|   stm32f427_437_429_439_lqfp208 IBIS Model
[IBIS ver]   4.2
[File name]  stm32f427_437_429_439_lqfp208.ibs
[File Rev]   1.3
[Date]   05-30-2014
[Source] Data Created at STMicroelectronics
[Notes]   File originated from ELDO simulations.
[Disclaimer]  This information is for modeling purpose only and is
   not guaranted. The information is subject to change without
   notice.
[Copyright] Copyright 2014 STMicroelectronics Inc.
[Component] stm32f427_437_429_439_lqfp208
[Manufacturer] STMicroelectronics
[Package]
| variable   typ   min   max
R_pkg   0.0   NA   NA
L_pkg   0.0H   NA   NA
C_pkg   0.0F   NA   NA
[Pin]   signal_name   model_name   R_pin   L_pin   C_pin
1   PE2   io8p_arsudq_ft   282.4E-3   13.6E-9   386.2E-15
2   PE3   io8p_arsudq_ft   277.3E-3   13.3E-9   362.7E-15
3   PE4   io8p_arsudq_ft   272.4E-3   13.0E-9   340.3E-15
4   PE5   io8p_arsudq_ft   267.8E-3   12.7E-9   318.8E-15
5   PE6   io8p_arsudq_ft   263.3E-3   12.4E-9   298.2E-15
6   VBAT   POWER   259.0E-3   12.1E-9   278.6E-15
7   PI8   io8p_arsudq_ft_v33   254.9E-3   11.9E-9   260.0E-15
8   PC13   io8p_arwsudq_ft_v33   251.1E-3   11.6E-9   242.3E-15
9   PC14   io8p_arwsudq_ft   247.4E-3   11.4E-9   225.6E-15
10   PC15   io8p_arsudq_ft   244.0E-3   11.2E-9   209.8E-15
11   PI9   io8p_arsudq_ft   240.8E-3   11.0E-9   195.0E-15
12   PI10   io8p_arsudq_ft   237.8E-3   10.8E-9   181.1E-15
13   PI11   io8p_arsudq_ft   234.9E-3   10.6E-9   168.2E-15
14   VSS   GND   232.3E-3   10.5E-9   156.3E-15
15   VDD   POWER   229.9E-3   10.3E-9   145.3E-15
16   PF0   io8p_arsudq_i2cin_ft   227.8E-3   10.2E-9   135.3E-15
17   PF1   io8p_arsudq_i2cin_ft   225.8E-3   10.1E-9   126.2E-15
18   PF2   io8p_arsudq_ft   224.0E-3   9.9E-9   118.1E-15
19   PI12   io8p_arsudq_ft   222.4E-3   9.9E-9   110.9E-15
20   PI13   io8p_arsudq_ft   221.1E-3   9.8E-9   104.7E-15
21   PI14   io8p_arsudq_ft   219.9E-3   9.7E-9   99.4E-15
22   PF3   io8p_arwsudq_ft   219.0E-3   9.6E-9   95.1E-15
23   PF4   io8p_arwsudq_ft   218.3E-3   9.6E-9   91.8E-15
24   PF5   io8p_arwsudq_ft   217.8E-3   9.6E-9   89.4E-15
25   VSS   GND   217.4E-3   9.5E-9   87.9E-15
26   VDD   POWER   217.3E-3   9.5E-9   87.5E-15
27   PF6   io8p_arwsudq_ft   217.3E-3   9.5E-9   87.5E-15
28   PF7   io8p_arwsudq_ft   217.4E-3   9.5E-9   87.9E-15
29   PF8   io8p_arwsudq_ft   217.8E-3   9.6E-9   89.4E-15
30   PF9   io8p_arwsudq_ft   218.3E-3   9.6E-9   91.8E-15
31   PF10   io8p_arwsudq_ft   219.0E-3   9.6E-9   95.1E-15
32   PH0   io8p_arsudq_ft   219.9E-3   9.7E-9   99.4E-15
33   PH1   io8p_arsudq_ft   221.1E-3   9.8E-9   104.7E-15
34   NRST   ioreset_ft_v33   222.4E-3   9.9E-9   110.9E-15
35   PC0   io8p_ar3wsudq_ft   224.0E-3   9.9E-9   118.1E-15
36   PC1   io8p_ar3wsudq_ft   225.8E-3   10.1E-9   126.2E-15
37   PC2   io8p_ar3wsudq_ft   227.8E-3   10.2E-9   135.3E-15
38   PC3   io8p_ar3wsudq_ft   229.9E-3   10.3E-9   145.3E-15
39   VDD   POWER   232.3E-3   10.5E-9   156.3E-15
40   VREFM   POWER   234.9E-3   10.6E-9   168.2E-15
41   VREFP   POWER   237.8E-3   10.8E-9   181.1E-15
42   VDDA   POWER   240.8E-3   11.0E-9   195.0E-15
43   PA0   io8p_ar3wsudq_ft_v33   244.0E-3   11.2E-9   209.8E-15
44   PA1   io8p_ar3wsudq_ft   247.4E-3   11.4E-9   225.6E-15
45   PA2   io8p_ar3wsudq_ft   251.1E-3   11.6E-9   242.3E-15
46   PH2   io8p_arsudq_ft   254.9E-3   11.9E-9   260.0E-15
47   PH3   io8p_arsudq_ft   259.0E-3   12.1E-9   278.6E-15
48   PH4   io8p_arsudq_i2cin_ft   263.3E-3   12.4E-9   298.2E-15
49   PH5   io8p_arsudq_i2cin_ft   267.8E-3   12.7E-9   318.8E-15
50   PA3   io8p_ar3wsudq_ft   272.4E-3   13.0E-9   340.3E-15
51   VSS   GND   277.3E-3   13.3E-9   362.7E-15
52   VDD   POWER   282.4E-3   13.6E-9   386.2E-15
53   PA4   io8p_ar3wsudq_ft   282.4E-3   13.6E-9   386.2E-15
54   PA5   io8p_ar3wsudq_ft   277.3E-3   13.3E-9   362.7E-15
55   PA6   io8p_ar3wsudq_ft   272.4E-3   13.0E-9   340.3E-15
56   PA7   io8p_ar3wsudq_ft   267.8E-3   12.7E-9   318.8E-15
57   PC4   io8p_ar3wsudq_ft   263.3E-3   12.4E-9   298.2E-15
58   PC5   io8p_ar3wsudq_ft   259.0E-3   12.1E-9   278.6E-15
59   VDD   POWER   254.9E-3   11.9E-9   260.0E-15
60   VSS   GND   251.1E-3   11.6E-9   242.3E-15
61   PB0   io8p_ar3wsudq_ft   247.4E-3   11.4E-9   225.6E-15
62   PB1   io8p_ar3wsudq_ft   244.0E-3   11.2E-9   209.8E-15
63   PB2   io8p_ar3wsudq_ft   240.8E-3   11.0E-9   195.0E-15
64   PI15   io8p_arsudq_ft   237.8E-3   10.8E-9   181.1E-15
65   PJ0   io8p_arsudq_ft   234.9E-3   10.6E-9   168.2E-15
66   PJ1   io8p_arsudq_ft   232.3E-3   10.5E-9   156.3E-15
67   PJ2   io8p_arsudq_ft   229.9E-3   10.3E-9   145.3E-15
68   PJ3   io8p_arsudq_ft   227.8E-3   10.2E-9   135.3E-15
69   PJ4   io8p_arsudq_ft   225.8E-3   10.1E-9   126.2E-15
70   PF11   io8p_arsudq_ft   224.0E-3   9.9E-9   118.1E-15
71   PF12   io8p_arsudq_ft   222.4E-3   9.9E-9   110.9E-15
72   VSS   GND   221.1E-3   9.8E-9   104.7E-15
73   VDD   POWER   219.9E-3   9.7E-9   99.4E-15
74   PF13   io8p_arsudq_ft   219.0E-3   9.6E-9   95.1E-15
75   PF14   io8p_arsudq_ft   218.3E-3   9.6E-9   91.8E-15
76   PF15   io8p_arsudq_ft   217.8E-3   9.6E-9   89.4E-15
77   PG0   io8p_arsudq_ft   217.4E-3   9.5E-9   87.9E-15
78   PG1   io8p_arsudq_ft   217.3E-3   9.5E-9   87.5E-15
79   PE7   io8p_arsudq_ft   217.3E-3   9.5E-9   87.5E-15
80   PE8   io8p_arsudq_ft   217.4E-3   9.5E-9   87.9E-15
81   PE9   io8p_arsudq_ft   217.8E-3   9.6E-9   89.4E-15
82   VSS   GND   218.3E-3   9.6E-9   91.8E-15
83   VDD   POWER   219.0E-3   9.6E-9   95.1E-15
84   PE10   io8p_arsudq_ft   219.9E-3   9.7E-9   99.4E-15
85   PE11   io8p_arsudq_ft   221.1E-3   9.8E-9   104.7E-15
86   PE12   io8p_arsudq_ft   222.4E-3   9.9E-9   110.9E-15
87   PE13   io8p_arsudq_ft   224.0E-3   9.9E-9   118.1E-15
88   PE14   io8p_arsudq_ft   225.8E-3   10.1E-9   126.2E-15
89   PE15   io8p_ar3wsudq_ft   227.8E-3   10.2E-9   135.3E-15
90   PB10   io8p_arsudq_i2cin_ft   229.9E-3   10.3E-9   145.3E-15
91   PB11   io8p_arsudq_i2cin_ft   232.3E-3   10.5E-9   156.3E-15
92   VCAP1   POWER   234.9E-3   10.6E-9   168.2E-15
93   VSS   GND   237.8E-3   10.8E-9   181.1E-15
94   VDD   POWER   240.8E-3   11.0E-9   195.0E-15
95   PJ5   io8p_arsudq_ft   244.0E-3   11.2E-9   209.8E-15
96   PH6   io8p_arsudq_ft   247.4E-3   11.4E-9   225.6E-15
97   PH7   io8p_arsudq_i2cin_ft   251.1E-3   11.6E-9   242.3E-15
98   PH8   io8p_arsudq_i2cin_ft   254.9E-3   11.9E-9   260.0E-15
99   PH9   io8p_arsudq_ft   259.0E-3   12.1E-9   278.6E-15
100   PH10   io8p_arsudq_ft   263.3E-3   12.4E-9   298.2E-15
101   PH11   io8p_arsudq_ft   267.8E-3   12.7E-9   318.8E-15
102   PH12   io8p_arsudq_ft   272.4E-3   13.0E-9   340.3E-15
103   VDD   POWER   277.3E-3   13.3E-9   362.7E-15
104   PB12   io8usb_id_otg_ft   282.4E-3   13.6E-9   386.2E-15
105   PB13   io8usb_vbus_otg_ft   282.4E-3   13.6E-9   386.2E-15
106   PB14   io8usb_lsfs_otg_ft   277.3E-3   13.3E-9   362.7E-15
107   PB15   io8usb_lsfs_otg_ft   272.4E-3   13.0E-9   340.3E-15
108   PD8   io8p_arsudq_ft   267.8E-3   12.7E-9   318.8E-15
109   PD9   io8p_arsudq_ft   263.3E-3   12.4E-9   298.2E-15
110   PD10   io8p_arsudq_ft   259.0E-3   12.1E-9   278.6E-15
111   PD11   io8p_arsudq_ft   254.9E-3   11.9E-9   260.0E-15
112   PD12   io8p_arsudq_ft   251.1E-3   11.6E-9   242.3E-15
113   PD13   io8p_arsudq_ft   247.4E-3   11.4E-9   225.6E-15
114   VSS   GND   244.0E-3   11.2E-9   209.8E-15
115   VDD   POWER   240.8E-3   11.0E-9   195.0E-15
116   PD14   io8p_arsudq_ft   237.8E-3   10.8E-9   181.1E-15
117   PD15   io8p_arsudq_ft   234.9E-3   10.6E-9   168.2E-15
118   PJ6   io8p_arsudq_ft   232.3E-3   10.5E-9   156.3E-15
119   PJ7   io8p_arsudq_ft   229.9E-3   10.3E-9   145.3E-15
120   PJ8   io8p_arsudq_ft   227.8E-3   10.2E-9   135.3E-15
121   PJ9   io8p_arsudq_ft   225.8E-3   10.1E-9   126.2E-15
122   PJ10   io8p_arsudq_ft   224.0E-3   9.9E-9   118.1E-15
123   PJ11   io8p_arsudq_ft   222.4E-3   9.9E-9   110.9E-15
124   VDD   POWER   221.1E-3   9.8E-9   104.7E-15
125   VSS   GND   219.9E-3   9.7E-9   99.4E-15
126   PK0   io8p_arsudq_ft   219.0E-3   9.6E-9   95.1E-15
127   PK1   io8p_arsudq_ft   218.3E-3   9.6E-9   91.8E-15
128   PK2   io8p_arsudq_ft   217.8E-3   9.6E-9   89.4E-15
129   PG2   io8p_arsudq_ft   217.4E-3   9.5E-9   87.9E-15
130   PG3   io8p_arsudq_ft   217.3E-3   9.5E-9   87.5E-15
131   PG4   io8p_arsudq_ft   217.3E-3   9.5E-9   87.5E-15
132   PG5   io8p_arsudq_ft   217.4E-3   9.5E-9   87.9E-15
133   PG6   io8p_arsudq_ft   217.8E-3   9.6E-9   89.4E-15
134   PG7   io8p_arsudq_ft   218.3E-3   9.6E-9   91.8E-15
135   PG8   io8p_arsudq_ft   219.0E-3   9.6E-9   95.1E-15
136   VSS   GND   219.9E-3   9.7E-9   99.4E-15
137   VDD   POWER   221.1E-3   9.8E-9   104.7E-15
138   PC6   io8p_arsudq_ft   222.4E-3   9.9E-9   110.9E-15
139   PC7   io8p_arsudq_ft   224.0E-3   9.9E-9   118.1E-15
140   PC8   io8p_arsudq_ft   225.8E-3   10.1E-9   126.2E-15
141   PC9   io8p_arsudq_i2cin_ft   227.8E-3   10.2E-9   135.3E-15
142   PA8   io8p_arsudq_i2cin_ft   229.9E-3   10.3E-9   145.3E-15
143   PA9   io8usb_vbus_otg_ft   232.3E-3   10.5E-9   156.3E-15
144   PA10   io8usb_id_otg_ft   234.9E-3   10.6E-9   168.2E-15
145   PA11   io8usb_lsfs_otg_ft   237.8E-3   10.8E-9   181.1E-15
146   PA12   io8usb_lsfs_otg_ft   240.8E-3   11.0E-9   195.0E-15
147   PA13   io8p_arsudq_ft   244.0E-3   11.2E-9   209.8E-15
148   VCAP2   POWER   247.4E-3   11.4E-9   225.6E-15
149   VSS   GND   251.1E-3   11.6E-9   242.3E-15
150   VDD   POWER   254.9E-3   11.9E-9   260.0E-15
151   PH13   io8p_arsudq_ft   259.0E-3   12.1E-9   278.6E-15
152   PH14   io8p_arsudq_ft   263.3E-3   12.4E-9   298.2E-15
153   PH15   io8p_arsudq_ft   267.8E-3   12.7E-9   318.8E-15
154   PI0   io8p_arsudq_ft   272.4E-3   13.0E-9   340.3E-15
155   PI1   io8p_arsudq_ft   277.3E-3   13.3E-9   362.7E-15
156   PI2   io8p_arsudq_ft   282.4E-3   13.6E-9   386.2E-15
157   PI3   io8p_arsudq_ft   282.4E-3   13.6E-9   386.2E-15
158   VDD   POWER   277.3E-3   13.3E-9   362.7E-15
159   PA14   io8p_arsudq_ft   272.4E-3   13.0E-9   340.3E-15
160   PA15   io8p_arsudq_ft   267.8E-3   12.7E-9   318.8E-15
161   PC10   io8p_arsudq_ft   263.3E-3   12.4E-9   298.2E-15
162   PC11   io8p_arsudq_ft   259.0E-3   12.1E-9   278.6E-15
163   PC12   io8p_arsudq_ft   254.9E-3   11.9E-9   260.0E-15
164   PD0   io8p_arsudq_ft   251.1E-3   11.6E-9   242.3E-15
165   PD1   io8p_arsudq_ft   247.4E-3   11.4E-9   225.6E-15
166   PD2   io8p_arsudq_ft   244.0E-3   11.2E-9   209.8E-15
167   PD3   io8p_arsudq_ft   240.8E-3   11.0E-9   195.0E-15
168   PD4   io8p_arsudq_ft   237.8E-3   10.8E-9   181.1E-15
169   PD5   io8p_arsudq_ft   234.9E-3   10.6E-9   168.2E-15
170   VSS   GND   232.3E-3   10.5E-9   156.3E-15
171   VDD   POWER   229.9E-3   10.3E-9   145.3E-15
172   PD6   io8p_arsudq_ft   227.8E-3   10.2E-9   135.3E-15
173   PD7   io8p_arsudq_ft   225.8E-3   10.1E-9   126.2E-15
174   PJ12   io8p_arsudq_ft   224.0E-3   9.9E-9   118.1E-15
175   PJ13   io8p_arsudq_ft   222.4E-3   9.9E-9   110.9E-15
176   PJ14   io8p_arsudq_ft   221.1E-3   9.8E-9   104.7E-15
177   PJ15   io8p_arsudq_ft   219.9E-3   9.7E-9   99.4E-15
178   PG9   io8p_arsudq_ft   219.0E-3   9.6E-9   95.1E-15
179   PG10   io8p_arsudq_ft   218.3E-3   9.6E-9   91.8E-15
180   PG11   io8p_arsudq_ft   217.8E-3   9.6E-9   89.4E-15
181   PG12   io8p_arsudq_ft   217.4E-3   9.5E-9   87.9E-15
182   PG13   io8p_arsudq_ft   217.3E-3   9.5E-9   87.5E-15
183   PG14   io8p_arsudq_ft   217.3E-3   9.5E-9   87.5E-15
184   VSS   GND   217.4E-3   9.5E-9   87.9E-15
185   VDD   POWER   217.8E-3   9.6E-9   89.4E-15
186   PK3   io8p_arsudq_ft   218.3E-3   9.6E-9   91.8E-15
187   PK4   io8p_arsudq_ft   219.0E-3   9.6E-9   95.1E-15
188   PK5   io8p_arsudq_ft   219.9E-3   9.7E-9   99.4E-15
189   PK6   io8p_arsudq_ft   221.1E-3   9.8E-9   104.7E-15
190   PK7   io8p_arsudq_ft   222.4E-3   9.9E-9   110.9E-15
191   PG15   io8p_arsudq_ft   224.0E-3   9.9E-9   118.1E-15
192   PB3   io8p_arsudq_ft   225.8E-3   10.1E-9   126.2E-15
193   PB4   io8p_arsudq_ft   227.8E-3   10.2E-9   135.3E-15
194   PB5   io8p_ar3wsudq_ft   229.9E-3   10.3E-9   145.3E-15
195   PB6   io8p_arsudq_i2cin_ft   232.3E-3   10.5E-9   156.3E-15
196   PB7   io8p_arsudq_i2cin_ft   234.9E-3   10.6E-9   168.2E-15
197   BOOT0   vpp_test_hv   237.8E-3   10.8E-9   181.1E-15
198   PB8   io8p_arsudq_i2cin_ft   240.8E-3   11.0E-9   195.0E-15
199   PB9   io8p_arsudq_i2cin_ft   244.0E-3   11.2E-9   209.8E-15
200   PE0   io8p_arsudq_ft   247.4E-3   11.4E-9   225.6E-15
201   PE1   io8p_arsudq_ft   251.1E-3   11.6E-9   242.3E-15
202   VSS   GND   254.9E-3   11.9E-9   260.0E-15
203   PDR_ON   io8p_arsudq_ft_v33   259.0E-3   12.1E-9   278.6E-15
204   VDD   POWER   263.3E-3   12.4E-9   298.2E-15
205   PI4   io8p_arsudq_ft   267.8E-3   12.7E-9   318.8E-15
206   PI5   io8p_arsudq_ft   272.4E-3   13.0E-9   340.3E-15
207   PI6   io8p_arsudq_ft   277.3E-3   13.3E-9   362.7E-15
208   PI7   io8p_arsudq_ft   282.4E-3   13.6E-9   386.2E-15
[Diff Pin]   inv_pin   vdiff   tdelay_typ  tdelay_min  tdelay_max
106   107   200mV   NA   NA   NA
146   145   200mV   NA   NA   NA
[Model Selector] io8p_ar3wsudq_ft
io8p00_ar3wsudq_ft_pd_lv  "SPEED00 1P8V, PD=40kOhm"
io8p00_ar3wsudq_ft_pu_lv  "SPEED00 1P8V, PU=40kOhm"
io8p00_ar3wsudq_ft_lv  "SPEED00 1P8V"
io8p01_ar3wsudq_ft_pd_lv  "SPEED01 1P8V, PD=40kOhm"
io8p01_ar3wsudq_ft_pu_lv  "SPEED01 1P8V, PU=40kOhm"
io8p01_ar3wsudq_ft_lv  "SPEED01 1P8V"
io8p10_ar3wsudq_ft_pd_lv  "SPEED10 1P8V, PD=40kOhm"
io8p10_ar3wsudq_ft_pu_lv  "SPEED10 1P8V, PU=40kOhm"
io8p10_ar3wsudq_ft_lv  "SPEED10 1P8V"
io8p11_ar3wsudq_ft_pd_lv  "SPEED11 1P8V, PD=40kOhm"
io8p11_ar3wsudq_ft_pu_lv  "SPEED11 1P8V, PU=40kOhm"
io8p11_ar3wsudq_ft_lv  "SPEED11 1P8V"
io8p00_ar3wsudq_ft_pd  "SPEED00, PD=40kOhm"
io8p00_ar3wsudq_ft_pu  "SPEED00, PU=40kOhm"
io8p00_ar3wsudq_ft  "SPEED00"
io8p01_ar3wsudq_ft_pd  "SPEED01, PD=40kOhm"
io8p01_ar3wsudq_ft_pu  "SPEED01, PU=40kOhm"
io8p01_ar3wsudq_ft  "SPEED01"
io8p10_ar3wsudq_ft_pd  "SPEED10, PD=40kOhm"
io8p10_ar3wsudq_ft_pu  "SPEED10, PU=40kOhm"
io8p10_ar3wsudq_ft  "SPEED10"
io8p11_ar3wsudq_ft_pd  "SPEED11, PD=40kOhm"
io8p11_ar3wsudq_ft_pu  "SPEED11, PU=40kOhm"
io8p11_ar3wsudq_ft  "SPEED11"
[Model Selector] io8p_ar3wsudq_ft_v33
io8p00_ar3wsudq_ft_v33_pd_lv  "SPEED00 1P8V, PD=40kOhm"
io8p00_ar3wsudq_ft_v33_pu_lv  "SPEED00 1P8V, PU=40kOhm"
io8p00_ar3wsudq_ft_v33_lv  "SPEED00 1P8V"
io8p01_ar3wsudq_ft_v33_pd_lv  "SPEED01 1P8V, PD=40kOhm"
io8p01_ar3wsudq_ft_v33_pu_lv  "SPEED01 1P8V, PU=40kOhm"
io8p01_ar3wsudq_ft_v33_lv  "SPEED01 1P8V"
io8p10_ar3wsudq_ft_v33_pd_lv  "SPEED10 1P8V, PD=40kOhm"
io8p10_ar3wsudq_ft_v33_pu_lv  "SPEED10 1P8V, PU=40kOhm"
io8p10_ar3wsudq_ft_v33_lv  "SPEED10 1P8V"
io8p11_ar3wsudq_ft_v33_pd_lv  "SPEED11 1P8V, PD=40kOhm"
io8p11_ar3wsudq_ft_v33_pu_lv  "SPEED11 1P8V, PU=40kOhm"
io8p11_ar3wsudq_ft_v33_lv  "SPEED11 1P8V"
io8p00_ar3wsudq_ft_v33_pd  "SPEED00, PD=40kOhm"
io8p00_ar3wsudq_ft_v33_pu  "SPEED00, PU=40kOhm"
io8p00_ar3wsudq_ft_v33  "SPEED00"
io8p01_ar3wsudq_ft_v33_pd  "SPEED01, PD=40kOhm"
io8p01_ar3wsudq_ft_v33_pu  "SPEED01, PU=40kOhm"
io8p01_ar3wsudq_ft_v33  "SPEED01"
io8p10_ar3wsudq_ft_v33_pd  "SPEED10, PD=40kOhm"
io8p10_ar3wsudq_ft_v33_pu  "SPEED10, PU=40kOhm"
io8p10_ar3wsudq_ft_v33  "SPEED10"
io8p11_ar3wsudq_ft_v33_pd  "SPEED11, PD=40kOhm"
io8p11_ar3wsudq_ft_v33_pu  "SPEED11, PU=40kOhm"
io8p11_ar3wsudq_ft_v33  "SPEED11"
[Model Selector] io8p_arsudq_ft
io8p00_arsudq_ft_pd_lv  "SPEED00 1P8V, PD=40kOhm"
io8p00_arsudq_ft_pu_lv  "SPEED00 1P8V, PU=40kOhm"
io8p00_arsudq_ft_lv  "SPEED00 1P8V"
io8p01_arsudq_ft_pd_lv  "SPEED01 1P8V, PD=40kOhm"
io8p01_arsudq_ft_pu_lv  "SPEED01 1P8V, PU=40kOhm"
io8p01_arsudq_ft_lv  "SPEED01 1P8V"
io8p10_arsudq_ft_pd_lv  "SPEED10 1P8V, PD=40kOhm"
io8p10_arsudq_ft_pu_lv  "SPEED10 1P8V, PU=40kOhm"
io8p10_arsudq_ft_lv  "SPEED10 1P8V"
io8p11_arsudq_ft_pd_lv  "SPEED11 1P8V, PD=40kOhm"
io8p11_arsudq_ft_pu_lv  "SPEED11 1P8V, PU=40kOhm"
io8p11_arsudq_ft_lv  "SPEED11 1P8V"
io8p00_arsudq_ft_pd  "SPEED00, PD=40kOhm"
io8p00_arsudq_ft_pu  "SPEED00, PU=40kOhm"
io8p00_arsudq_ft  "SPEED00"
io8p01_arsudq_ft_pd  "SPEED01, PD=40kOhm"
io8p01_arsudq_ft_pu  "SPEED01, PU=40kOhm"
io8p01_arsudq_ft  "SPEED01"
io8p10_arsudq_ft_pd  "SPEED10, PD=40kOhm"
io8p10_arsudq_ft_pu  "SPEED10, PU=40kOhm"
io8p10_arsudq_ft  "SPEED10"
io8p11_arsudq_ft_pd  "SPEED11, PD=40kOhm"
io8p11_arsudq_ft_pu  "SPEED11, PU=40kOhm"
io8p11_arsudq_ft  "SPEED11"
[Model Selector] io8p_arsudq_ft_v33
io8p00_arsudq_ft_v33_pd_lv  "SPEED00 1P8V, PD=40kOhm"
io8p00_arsudq_ft_v33_pu_lv  "SPEED00 1P8V, PU=40kOhm"
io8p00_arsudq_ft_v33_lv  "SPEED00 1P8V"
io8p01_arsudq_ft_v33_pd_lv  "SPEED01 1P8V, PD=40kOhm"
io8p01_arsudq_ft_v33_pu_lv  "SPEED01 1P8V, PU=40kOhm"
io8p01_arsudq_ft_v33_lv  "SPEED01 1P8V"
io8p10_arsudq_ft_v33_pd_lv  "SPEED10 1P8V, PD=40kOhm"
io8p10_arsudq_ft_v33_pu_lv  "SPEED10 1P8V, PU=40kOhm"
io8p10_arsudq_ft_v33_lv  "SPEED10 1P8V"
io8p11_arsudq_ft_v33_pd_lv  "SPEED11 1P8V, PD=40kOhm"
io8p11_arsudq_ft_v33_pu_lv  "SPEED11 1P8V, PU=40kOhm"
io8p11_arsudq_ft_v33_lv  "SPEED11 1P8V"
io8p00_arsudq_ft_v33_pd  "SPEED00, PD=40kOhm"
io8p00_arsudq_ft_v33_pu  "SPEED00, PU=40kOhm"
io8p00_arsudq_ft_v33  "SPEED00"
io8p01_arsudq_ft_v33_pd  "SPEED01, PD=40kOhm"
io8p01_arsudq_ft_v33_pu  "SPEED01, PU=40kOhm"
io8p01_arsudq_ft_v33  "SPEED01"
io8p10_arsudq_ft_v33_pd  "SPEED10, PD=40kOhm"
io8p10_arsudq_ft_v33_pu  "SPEED10, PU=40kOhm"
io8p10_arsudq_ft_v33  "SPEED10"
io8p11_arsudq_ft_v33_pd  "SPEED11, PD=40kOhm"
io8p11_arsudq_ft_v33_pu  "SPEED11, PU=40kOhm"
io8p11_arsudq_ft_v33  "SPEED11"
[Model Selector] io8p_arsudq_i2cin_ft
io8p00_arsudq_i2cin_ft_pd_lv  "SPEED00 1P8V, PD=40kOhm"
io8p00_arsudq_i2cin_ft_pu_lv  "SPEED00 1P8V, PU=40kOhm"
io8p00_arsudq_i2cin_ft_lv  "SPEED00 1P8V"
io8p01_arsudq_i2cin_ft_pd_lv  "SPEED01 1P8V, PD=40kOhm"
io8p01_arsudq_i2cin_ft_pu_lv  "SPEED01 1P8V, PU=40kOhm"
io8p01_arsudq_i2cin_ft_lv  "SPEED01 1P8V"
io8p10_arsudq_i2cin_ft_pd_lv  "SPEED10 1P8V, PD=40kOhm"
io8p10_arsudq_i2cin_ft_pu_lv  "SPEED10 1P8V, PU=40kOhm"
io8p10_arsudq_i2cin_ft_lv  "SPEED10 1P8V"
io8p11_arsudq_i2cin_ft_pd_lv  "SPEED11 1P8V, PD=40kOhm"
io8p11_arsudq_i2cin_ft_pu_lv  "SPEED11 1P8V, PU=40kOhm"
io8p11_arsudq_i2cin_ft_lv  "SPEED11 1P8V"
io8p00_arsudq_i2cin_ft_pd  "SPEED00, PD=40kOhm"
io8p00_arsudq_i2cin_ft_pu  "SPEED00, PU=40kOhm"
io8p00_arsudq_i2cin_ft  "SPEED00"
io8p01_arsudq_i2cin_ft_pd  "SPEED01, PD=40kOhm"
io8p01_arsudq_i2cin_ft_pu  "SPEED01, PU=40kOhm"
io8p01_arsudq_i2cin_ft  "SPEED01"
io8p10_arsudq_i2cin_ft_pd  "SPEED10, PD=40kOhm"
io8p10_arsudq_i2cin_ft_pu  "SPEED10, PU=40kOhm"
io8p10_arsudq_i2cin_ft  "SPEED10"
io8p11_arsudq_i2cin_ft_pd  "SPEED11, PD=40kOhm"
io8p11_arsudq_i2cin_ft_pu  "SPEED11, PU=40kOhm"
io8p11_arsudq_i2cin_ft  "SPEED11"
[Model Selector] io8p_arwsudq_ft
io8p00_arwsudq_ft_pd_lv  "SPEED00 1P8V, PD=40kOhm"
io8p00_arwsudq_ft_pu_lv  "SPEED00 1P8V, PU=40kOhm"
io8p00_arwsudq_ft_lv  "SPEED00 1P8V"
io8p01_arwsudq_ft_pd_lv  "SPEED01 1P8V, PD=40kOhm"
io8p01_arwsudq_ft_pu_lv  "SPEED01 1P8V, PU=40kOhm"
io8p01_arwsudq_ft_lv  "SPEED01 1P8V"
io8p10_arwsudq_ft_pd_lv  "SPEED10 1P8V, PD=40kOhm"
io8p10_arwsudq_ft_pu_lv  "SPEED10 1P8V, PU=40kOhm"
io8p10_arwsudq_ft_lv  "SPEED10 1P8V"
io8p11_arwsudq_ft_pd_lv  "SPEED11 1P8V, PD=40kOhm"
io8p11_arwsudq_ft_pu_lv  "SPEED11 1P8V, PU=40kOhm"
io8p11_arwsudq_ft_lv  "SPEED11 1P8V"
io8p00_arwsudq_ft_pd  "SPEED00, PD=40kOhm"
io8p00_arwsudq_ft_pu  "SPEED00, PU=40kOhm"
io8p00_arwsudq_ft  "SPEED00"
io8p01_arwsudq_ft_pd  "SPEED01, PD=40kOhm"
io8p01_arwsudq_ft_pu  "SPEED01, PU=40kOhm"
io8p01_arwsudq_ft  "SPEED01"
io8p10_arwsudq_ft_pd  "SPEED10, PD=40kOhm"
io8p10_arwsudq_ft_pu  "SPEED10, PU=40kOhm"
io8p10_arwsudq_ft  "SPEED10"
io8p11_arwsudq_ft_pd  "SPEED11, PD=40kOhm"
io8p11_arwsudq_ft_pu  "SPEED11, PU=40kOhm"
io8p11_arwsudq_ft  "SPEED11"
[Model Selector] io8p_arwsudq_ft_v33
io8p00_arwsudq_ft_v33_pd_lv  "SPEED00 1P8V, PD=40kOhm"
io8p00_arwsudq_ft_v33_pu_lv  "SPEED00 1P8V, PU=40kOhm"
io8p00_arwsudq_ft_v33_lv  "SPEED00 1P8V"
io8p01_arwsudq_ft_v33_pd_lv  "SPEED01 1P8V, PD=40kOhm"
io8p01_arwsudq_ft_v33_pu_lv  "SPEED01 1P8V, PU=40kOhm"
io8p01_arwsudq_ft_v33_lv  "SPEED01 1P8V"
io8p10_arwsudq_ft_v33_pd_lv  "SPEED10 1P8V, PD=40kOhm"
io8p10_arwsudq_ft_v33_pu_lv  "SPEED10 1P8V, PU=40kOhm"
io8p10_arwsudq_ft_v33_lv  "SPEED10 1P8V"
io8p11_arwsudq_ft_v33_pd_lv  "SPEED11 1P8V, PD=40kOhm"
io8p11_arwsudq_ft_v33_pu_lv  "SPEED11 1P8V, PU=40kOhm"
io8p11_arwsudq_ft_v33_lv  "SPEED11 1P8V"
io8p00_arwsudq_ft_v33_pd  "SPEED00, PD=40kOhm"
io8p00_arwsudq_ft_v33_pu  "SPEED00, PU=40kOhm"
io8p00_arwsudq_ft_v33  "SPEED00"
io8p01_arwsudq_ft_v33_pd  "SPEED01, PD=40kOhm"
io8p01_arwsudq_ft_v33_pu  "SPEED01, PU=40kOhm"
io8p01_arwsudq_ft_v33  "SPEED01"
io8p10_arwsudq_ft_v33_pd  "SPEED10, PD=40kOhm"
io8p10_arwsudq_ft_v33_pu  "SPEED10, PU=40kOhm"
io8p10_arwsudq_ft_v33  "SPEED10"
io8p11_arwsudq_ft_v33_pd  "SPEED11, PD=40kOhm"
io8p11_arwsudq_ft_v33_pu  "SPEED11, PU=40kOhm"
io8p11_arwsudq_ft_v33  "SPEED11"
[Model Selector] io8usb_id_otg_ft
io8p00_id_otg_ft_pd_lv  "SPEED00 1P8V, PD=14kOhm"
io8p00_id_otg_ft_pu_lv  "SPEED00 1P8V, PU=14kOhm"
io8p00_id_otg_ft_lv  "SPEED00 1P8V"
io8p01_id_otg_ft_pd_lv  "SPEED01 1P8V, PD=14kOhm"
io8p01_id_otg_ft_pu_lv  "SPEED01 1P8V, PU=14kOhm"
io8p01_id_otg_ft_lv  "SPEED01 1P8V"
io8p10_id_otg_ft_pd_lv  "SPEED10 1P8V, PD=14kOhm"
io8p10_id_otg_ft_pu_lv  "SPEED10 1P8V, PU=14kOhm"
io8p10_id_otg_ft_lv  "SPEED10 1P8V"
io8p11_id_otg_ft_pd_lv  "SPEED11 1P8V, PD=14kOhm"
io8p11_id_otg_ft_pu_lv  "SPEED11 1P8V, PU=14kOhm"
io8p11_id_otg_ft_lv  "SPEED11 1P8V"
io8p00_id_otg_ft_pd  "SPEED00, PD=14kOhm"
io8p00_id_otg_ft_pu  "SPEED00, PU=14kOhm"
io8p00_id_otg_ft  "SPEED00"
io8p01_id_otg_ft_pd  "SPEED01, PD=14kOhm"
io8p01_id_otg_ft_pu  "SPEED01, PU=14kOhm"
io8p01_id_otg_ft  "SPEED01"
io8p10_id_otg_ft_pd  "SPEED10, PD=14kOhm"
io8p10_id_otg_ft_pu  "SPEED10, PU=14kOhm"
io8p10_id_otg_ft  "SPEED10"
io8p11_id_otg_ft_pd  "SPEED11, PD=14kOhm"
io8p11_id_otg_ft_pu  "SPEED11, PU=14kOhm"
io8p11_id_otg_ft  "SPEED11"
[Model Selector] io8usb_lsfs_otg_ft
io8usb_ls_otg_ft_dpdn_pd  "LS USB DP/DN IO + PD=20kOhm"
io8usb_ls_otg_ft_dpdn_pupu2  "LS USB DP/DN IO + PU/PU2=2.2kOhm"
io8usb_ls_otg_ft_dpdn_pu2  "LS USB DP/DN IO + PU2=1.2kOhm"
io8usb_ls_otg_ft_dpdn_pu  "LS USB DP/DN IO + PU=1.2kOhm"
io8usb_ls_otg_ft_dpdn  "LS USB DP/DN IO"
io8usb_fs_otg_ft_dpdn_pd  "HS USB DP/DN IO + PD=20kOhm"
io8usb_fs_otg_ft_dpdn_pupu2  "HS USB DP/DN IO + PU/PU2=2.2kOhm"
io8usb_fs_otg_ft_dpdn_pu2  "HS USB DP/DN IO + PU2=1.2kOhm"
io8usb_fs_otg_ft_dpdn_pu  "HS USB DP/DN IO + PU=1.2kOhm"
io8usb_fs_otg_ft_dpdn  "HS USB DP/DN IO"
io8p00_lsfs_otg_ft_pd_lv  "SPEED00 1P8V, PD=40kOhm"
io8p00_lsfs_otg_ft_pu_lv  "SPEED00 1P8V, PU=40kOhm"
io8p00_lsfs_otg_ft_lv  "SPEED00 1P8V"
io8p01_lsfs_otg_ft_pd_lv  "SPEED01 1P8V, PD=40kOhm"
io8p01_lsfs_otg_ft_pu_lv  "SPEED01 1P8V, PU=40kOhm"
io8p01_lsfs_otg_ft_lv  "SPEED01 1P8V"
io8p10_lsfs_otg_ft_pd_lv  "SPEED10 1P8V, PD=40kOhm"
io8p10_lsfs_otg_ft_pu_lv  "SPEED10 1P8V, PU=40kOhm"
io8p10_lsfs_otg_ft_lv  "SPEED10 1P8V"
io8p11_lsfs_otg_ft_pd_lv  "SPEED11 1P8V, PD=40kOhm"
io8p11_lsfs_otg_ft_pu_lv  "SPEED11 1P8V, PU=40kOhm"
io8p11_lsfs_otg_ft_lv  "SPEED11 1P8V"
io8p00_lsfs_otg_ft_pd  "SPEED00, PD=40kOhm"
io8p00_lsfs_otg_ft_pu  "SPEED00, PU=40kOhm"
io8p00_lsfs_otg_ft  "SPEED00"
io8p01_lsfs_otg_ft_pd  "SPEED01, PD=40kOhm"
io8p01_lsfs_otg_ft_pu  "SPEED01, PU=40kOhm"
io8p01_lsfs_otg_ft  "SPEED01"
io8p10_lsfs_otg_ft_pd  "SPEED10, PD=40kOhm"
io8p10_lsfs_otg_ft_pu  "SPEED10, PU=40kOhm"
io8p10_lsfs_otg_ft  "SPEED10"
io8p11_lsfs_otg_ft_pd  "SPEED11, PD=40kOhm"
io8p11_lsfs_otg_ft_pu  "SPEED11, PU=40kOhm"
io8p11_lsfs_otg_ft  "SPEED11"
[Model Selector] io8usb_vbus_otg_ft
io8psenb_vbus_otg_ft  "VBUS PULSE, SENSE VB"
io8psenab_vbus_otg_ft  "VBUS PULSE, SENSE VA and VB"
io8psena_vbus_otg_ft  "VBUS PULSE, SENSE VA"
io8psen_vbus_otg_ft  "VBUS PULSE"
io8p00_vbus_otg_ft_pd_lv  "SPEED00 1P8V, PD=40kOhm"
io8p00_vbus_otg_ft_pu_lv  "SPEED00 1P8V, PU=40kOhm"
io8p00_vbus_otg_ft_lv  "SPEED00 1P8V"
io8p01_vbus_otg_ft_pd_lv  "SPEED01 1P8V, PD=40kOhm"
io8p01_vbus_otg_ft_pu_lv  "SPEED01 1P8V, PU=40kOhm"
io8p01_vbus_otg_ft_lv  "SPEED01 1P8V"
io8p10_vbus_otg_ft_pd_lv  "SPEED10 1P8V, PD=40kOhm"
io8p10_vbus_otg_ft_pu_lv  "SPEED10 1P8V, PU=40kOhm"
io8p10_vbus_otg_ft_lv  "SPEED10 1P8V"
io8p11_vbus_otg_ft_pd_lv  "SPEED11 1P8V, PD=40kOhm"
io8p11_vbus_otg_ft_pu_lv  "SPEED11 1P8V, PU=40kOhm"
io8p11_vbus_otg_ft_lv  "SPEED11 1P8V"
io8p00_vbus_otg_ft_pd  "SPEED00, PD=40kOhm"
io8p00_vbus_otg_ft_pu  "SPEED00, PU=40kOhm"
io8p00_vbus_otg_ft  "SPEED00"
io8p01_vbus_otg_ft_pd  "SPEED01, PD=40kOhm"
io8p01_vbus_otg_ft_pu  "SPEED01, PU=40kOhm"
io8p01_vbus_otg_ft  "SPEED01"
io8p10_vbus_otg_ft_pd  "SPEED10, PD=40kOhm"
io8p10_vbus_otg_ft_pu  "SPEED10, PU=40kOhm"
io8p10_vbus_otg_ft  "SPEED10"
io8p11_vbus_otg_ft_pd  "SPEED11, PD=40kOhm"
io8p11_vbus_otg_ft_pu  "SPEED11, PU=40kOhm"
io8p11_vbus_otg_ft  "SPEED11"
[Model Selector] ioreset_ft_v33
ioreset_ft_v33_pu_lv  "ioreset 1P8V + PU=40kOhm"
ioreset_ft_v33_nopu_lv  "ioreset 1P8V"
ioreset_ft_v33_pu  "ioreset + PU=40kOhm"
ioreset_ft_v33_nopu  "ioreset"
[Model Selector] vpp_test_hv
vpp_test_hv_2p4  "Input Buffer 1P8V"
vpp_test_hv_3p3  "Input Buffer"
| Models and submodels in the file (260): io8p00_ar3wsudq_ft_pd_lv (I/O), io8p00_ar3wsudq_ft_pu_lv (I/O), io8p00_ar3wsudq_ft_lv (I/O), io8p01_ar3wsudq_ft_pd_lv (I/O), io8p01_ar3wsudq_ft_pu_lv (I/O), io8p01_ar3wsudq_ft_lv (I/O), io8p10_ar3wsudq_ft_pd_lv (I/O), io8p10_ar3wsudq_ft_pu_lv (I/O), io8p10_ar3wsudq_ft_lv (I/O), io8p11_ar3wsudq_ft_pd_lv (I/O), io8p11_ar3wsudq_ft_pu_lv (I/O), io8p11_ar3wsudq_ft_lv (I/O), io8p00_ar3wsudq_ft_pd (I/O), io8p00_ar3wsudq_ft_pu (I/O), io8p00_ar3wsudq_ft (I/O), io8p01_ar3wsudq_ft_pd (I/O), io8p01_ar3wsudq_ft_pu (I/O), io8p01_ar3wsudq_ft (I/O), io8p10_ar3wsudq_ft_pd (I/O), io8p10_ar3wsudq_ft_pu (I/O), io8p10_ar3wsudq_ft (I/O), io8p11_ar3wsudq_ft_pd (I/O), io8p11_ar3wsudq_ft_pu (I/O), io8p11_ar3wsudq_ft (I/O), io8p00_ar3wsudq_ft_v33_pd_lv (I/O), io8p00_ar3wsudq_ft_v33_pu_lv (I/O), io8p00_ar3wsudq_ft_v33_lv (I/O), io8p01_ar3wsudq_ft_v33_pd_lv (I/O), io8p01_ar3wsudq_ft_v33_pu_lv (I/O), io8p01_ar3wsudq_ft_v33_lv (I/O), io8p10_ar3wsudq_ft_v33_pd_lv (I/O), io8p10_ar3wsudq_ft_v33_pu_lv (I/O), io8p10_ar3wsudq_ft_v33_lv (I/O), io8p11_ar3wsudq_ft_v33_pd_lv (I/O), io8p11_ar3wsudq_ft_v33_pu_lv (I/O), io8p11_ar3wsudq_ft_v33_lv (I/O), io8p00_ar3wsudq_ft_v33_pd (I/O), io8p00_ar3wsudq_ft_v33_pu (I/O), io8p00_ar3wsudq_ft_v33 (I/O), io8p01_ar3wsudq_ft_v33_pd (I/O), io8p01_ar3wsudq_ft_v33_pu (I/O), io8p01_ar3wsudq_ft_v33 (I/O), io8p10_ar3wsudq_ft_v33_pd (I/O), io8p10_ar3wsudq_ft_v33_pu (I/O), io8p10_ar3wsudq_ft_v33 (I/O), io8p11_ar3wsudq_ft_v33_pd (I/O), io8p11_ar3wsudq_ft_v33_pu (I/O), io8p11_ar3wsudq_ft_v33 (I/O), io8p00_arsudq_ft_pd_lv (I/O), io8p00_arsudq_ft_pu_lv (I/O), io8p00_arsudq_ft_lv (I/O), io8p01_arsudq_ft_pd_lv (I/O), io8p01_arsudq_ft_pu_lv (I/O), io8p01_arsudq_ft_lv (I/O), io8p10_arsudq_ft_pd_lv (I/O), io8p10_arsudq_ft_pu_lv (I/O), io8p10_arsudq_ft_lv (I/O), io8p11_arsudq_ft_pd_lv (I/O), io8p11_arsudq_ft_pu_lv (I/O), io8p11_arsudq_ft_lv (I/O), io8p00_arsudq_ft_pd (I/O), io8p00_arsudq_ft_pu (I/O), io8p00_arsudq_ft (I/O), io8p01_arsudq_ft_pd (I/O), io8p01_arsudq_ft_pu (I/O), io8p01_arsudq_ft (I/O), io8p10_arsudq_ft_pd (I/O), io8p10_arsudq_ft_pu (I/O), io8p10_arsudq_ft (I/O), io8p11_arsudq_ft_pd (I/O), io8p11_arsudq_ft_pu (I/O), io8p11_arsudq_ft (I/O), io8p00_arsudq_ft_v33_pd_lv (I/O), io8p00_arsudq_ft_v33_pu_lv (I/O), io8p00_arsudq_ft_v33_lv (I/O), io8p01_arsudq_ft_v33_pd_lv (I/O), io8p01_arsudq_ft_v33_pu_lv (I/O), io8p01_arsudq_ft_v33_lv (I/O), io8p10_arsudq_ft_v33_pd_lv (I/O), io8p10_arsudq_ft_v33_pu_lv (I/O)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
